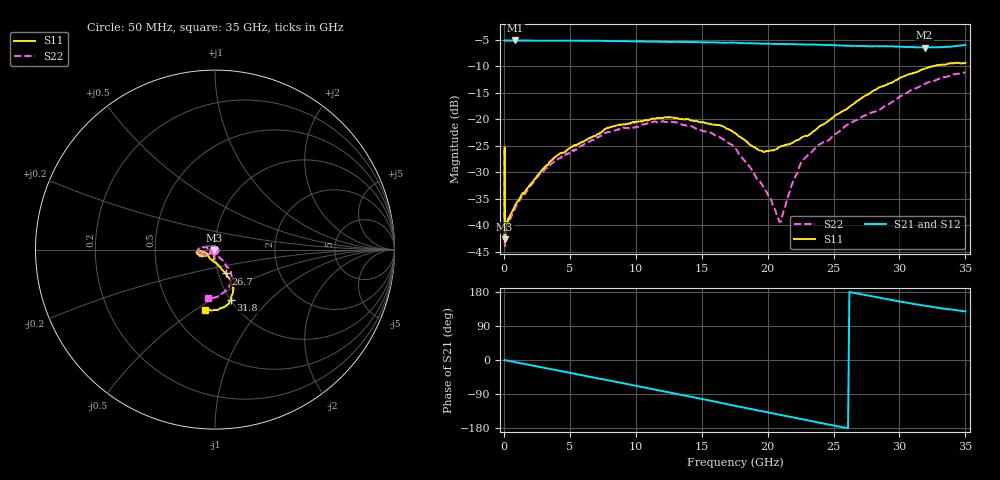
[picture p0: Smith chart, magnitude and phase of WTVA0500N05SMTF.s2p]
! 50 ohm 2-Port S-parameters measured by Modelithics Inc support@modelithics.com  Tampa, FL USA 813-866-6335 (February 2024)
! Smiths Interconnect,  5dB P/N: WTVA0500N05SMTF, Temperature: 25C
! Board: 10 mil Rogers 4350B, Mounting Pad Dimensions: Length: 15 mils, Width: 25 mils, Gap: 40 mils.
# Hz S MA R 50
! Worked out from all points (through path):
!   486 points, 50 MHz to 35 GHz, reference 50 ohm
!   highest |S21| = -5.16 dB at 850 MHz (marker M1); lowest = -6.5 dB at 31.9 GHz (marker M2)
!   group delay of S21, straight-line fit = 19 ps
!   lowest |S11| = -42.7 dB at 50 MHz (marker M3), VSWR 1.01, Z = 49.3 - j0.306 ohm
!   |S11| at or under -10 dB: start of sweep to 32.57 GHz
!   |S22| runs from -44.0 to -11.2 dB; largest |S21 - S12| = 0.011
!   S11 on the Smith chart (normalised r, x): 50 MHz: 0.99, -0.01; 26.7 GHz: 1.08, -0.29; 31.8 GHz: 1.00, -0.62; 35 GHz: 0.72, -0.54
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5e7  0.00733 -155.0  0.5506 -0.3  0.5502 -0.4  0.007266 -175.2
8e7  0.008288 -154.5  0.5503 -0.4  0.5495 -0.5  0.006319 -174.1
9e7  0.01069 -172.2  0.5505 -0.6  0.5502 -0.6  0.009222 -171.0
1.7e8  0.01021 -162.6  0.5505 -1.1  0.5503 -1.1  0.009442 -162.1
8.5e8  0.01543 -147.6  0.5521 -5.5  0.5525 -5.6  0.01449 -144.6
2.75e9  0.03158 -140.7  0.55 -18.3  0.5497 -18.3  0.03052 -140.8
3.95e9  0.0446 -143.0  0.5496 -26.4  0.5492 -26.4  0.04031 -145.3
5.9e9  0.06076 -146.8  0.549 -39.7  0.5489 -39.7  0.05635 -150.2
7.9e9  0.08285 -154.0  0.5454 -53.5  0.5453 -53.5  0.07584 -160.7
1.17e10  0.1024 -168.3  0.5378 -79.7  0.5376 -79.7  0.09425 -174.8
1.57e10  0.08939 -173.3  0.529 -107.5  0.5289 -107.7  0.0744 170.7
1.76e10  0.07281 -170.8  0.526 -121.5  0.5259 -121.3  0.05224 166.2
1.95e10  0.05053 -152.4  0.5156 -134.7  0.5154 -134.6  0.02482 -170.1
2.09e10  0.05461 -125.6  0.511 -144.3  0.5108 -144.2  0.01072 -116.7
2.11e10  0.0557 -123.2  0.5108 -145.6  0.5104 -145.5  0.01207 -95.2
2.25e10  0.06599 -98.3  0.5064 -155.6  0.5067 -155.3  0.03793 -60.6
2.34e10  0.07534 -84.5  0.505 -161.7  0.5052 -161.5  0.04965 -59.5
2.67e10  0.1453 -66.1  0.4915 176.1  0.4914 176.3  0.0976 -55.5
2.92e10  0.2154 -64.0  0.486 159.7  0.4858 160.2  0.1386 -54.1
3.18e10  0.2962 -72.7  0.4752 143.6  0.4752 144.6  0.2114 -65.9
3.19e10  0.298 -73.4  0.4736 143.0  0.4738 144.1  0.2139 -66.9
3.5e10  0.3389 -99.9  0.502 128.3  0.5017 128.6  0.2751 -98.6
